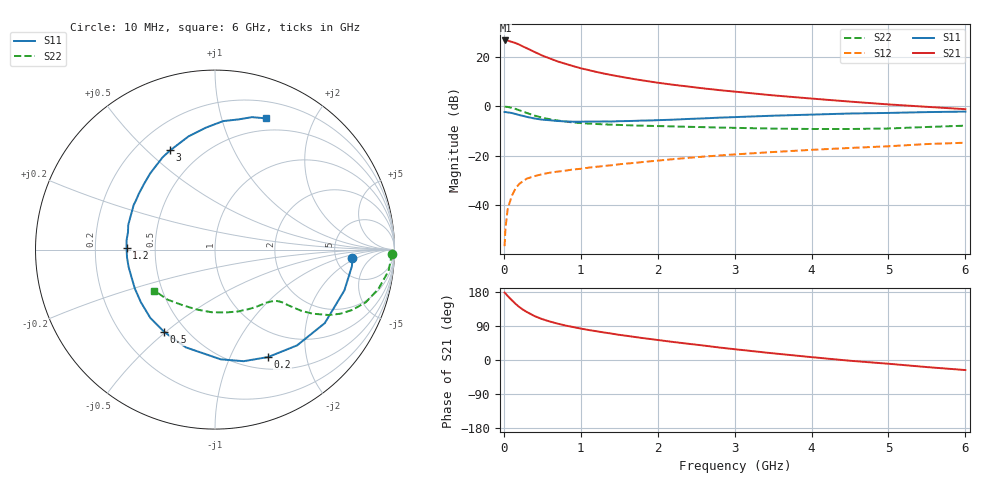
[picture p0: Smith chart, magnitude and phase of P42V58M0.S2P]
! SIEMENS Small Signal Semiconductors
! BFP182
! Si NPN RF Bipolar Junction Transistor in SOT143
! VCE = 2.5 V  IC = 8 mA
! Common Emitter S-Parameters:  March  1996
# GHz  S  MA  R  50
!  f  S11  S21  S12  S22
! GHz  MAG  ANG  MAG  ANG  MAG  ANG  MAG  ANG
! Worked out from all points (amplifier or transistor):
!   36 points, 10 MHz to 6 GHz, reference 50 ohm
!   highest |S21| = 26.6 dB at 20 MHz (marker M1)
!   |S21| within 3 dB of that: start of sweep to 288.2 MHz
!   unconditionally stable (mu >= 1): 1.28 GHz to 5.395 GHz
!   at 250 MHz: K = 0.29, MSG = 27.2 dB, |S12| = -30.2 dB
!   at 1.4 GHz: K = 1.05, MAG = 16.9 dB, |S12| = -23.8 dB
!   at 6 GHz: K = 0.94, MSG = 6.8 dB, |S12| = -14.7 dB
!   lowest NFmin = 1.40 dB at 450 MHz
!   S11 on the Smith chart (normalised r, x): 10 MHz: 7.22, -1.60; 200 MHz: 0.65, -1.40; 500 MHz: 0.38, -0.49; 1.2 GHz: 0.34, +0.01; 3 GHz: 0.34, +0.59; 6 GHz: 0.37, +1.40
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0.01  0.767 -3.4  21.25 177.8  0.0015 90.3  0.9861 -1.3
0.02  0.7685 -6.9  21.45 175.9  0.0033 82.3  0.9825 -2.7
0.05  0.7559 -17.5  21.31 168.8  0.0084 84.1  0.9744 -7.0
0.1  0.7362 -33.8  20.17 158.5  0.0151 73.4  0.9365 -13.5
0.15  0.7028 -49.4  19.07 148.6  0.0218 66.3  0.8906 -19.2
0.2  0.6678 -63.7  17.72 140.0  0.0271 60.9  0.836 -23.7
0.25  0.6419 -75.6  16.14 132.7  0.031 56.4  0.7842 -27.1
0.3  0.6123 -87.0  14.9 126.6  0.0348 52.7  0.7337 -29.8
0.4  0.5685 -106.6  12.55 115.8  0.039 47.7  0.6505 -33.3
0.5  0.5392 -121.6  10.62 107.8  0.0427 43.9  0.5907 -35.3
0.6  0.524 -133.5  9.259 101.4  0.0458 42.4  0.5492 -36.3
0.7  0.5066 -144.5  8.087 95.9  0.0481 41.5  0.5171 -37.1
0.9  0.4902 -161.2  6.52 87.0  0.0531 40.8  0.4733 -38.2
1.1  0.4922 -174.9  5.415 79.2  0.0578 41.0  0.449 -39.7
1.2  0.4929 178.8  4.976 76.0  0.0601 40.6  0.4404 -40.6
1.7  0.5094 155.3  3.542 60.9  0.0721 41.2  0.4106 -46.1
2.2  0.5387 137.2  2.733 47.6  0.0857 40.4  0.394 -53.7
3  0.6068 114.3  1.987 28.5  0.107 36.5  0.3683 -69.3
3.5  0.648 103.1  1.669 17.6  0.1196 33.3  0.3553 -80.7
4.5  0.7174 86.4  1.248 -2.0  0.1445 26.7  0.3488 -106.7
5.5  0.7662 74.4  0.979 -18.7  0.1734 19.8  0.3834 -133.2
6  0.7842 68.8  0.877 -26.5  0.1844 15.2  0.4076 -145.8
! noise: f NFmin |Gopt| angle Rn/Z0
0.45  1.4  0.26  41  0.29
0.9  1.5  0.25  83  0.23
1.8  2  0.21  162  0.2
